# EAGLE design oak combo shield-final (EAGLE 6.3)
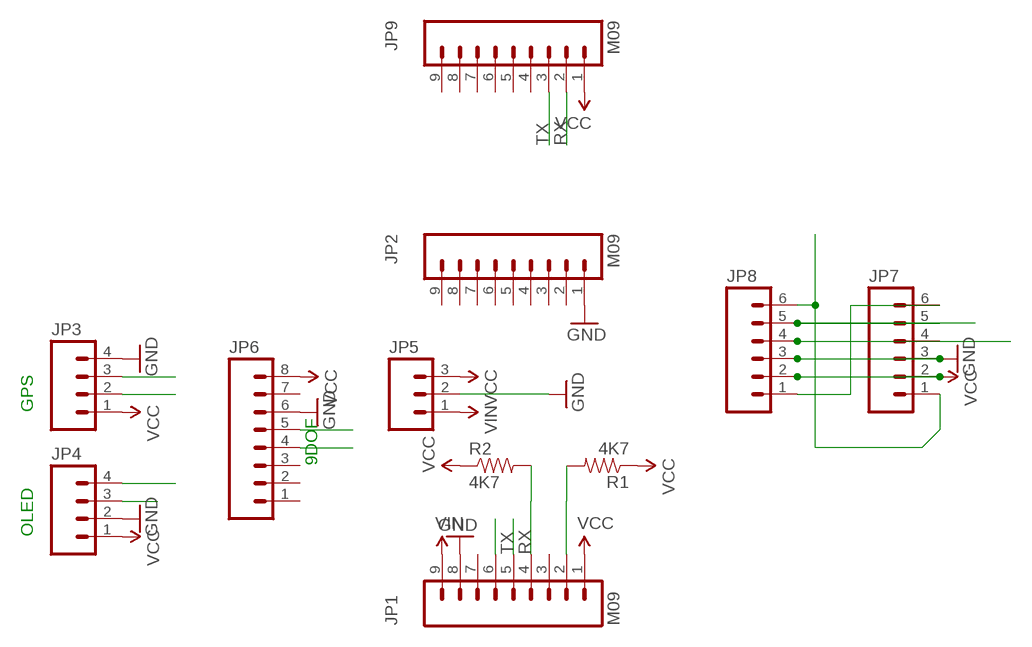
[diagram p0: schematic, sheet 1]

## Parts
JP1  M09  [1X09]
JP2  M09  [1X09]
JP3  M04PTH  [1X04]
JP4  M04PTH  [1X04]
JP5  M03PTH  [1X03]
JP6  M081X08  [1X08]
JP7  M06LOCK  [1X06_LOCK]
JP8  M06LOCK  [1X06_LOCK]
JP9  M09  [1X09]
R1  4K7  RESISTORPTH-1/4W  [AXIAL-0.4]
R2  4K7  RESISTORPTH-1/4W  [AXIAL-0.4]

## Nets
GND [POWER]: JP1.8 JP2.1 JP3.4 JP4.2 JP5.2 JP6.6 JP7.3 JP8.3
RX: JP1.5 JP3.3 JP7.4 JP8.4 JP9.2
SCL: JP1.4 JP4.3 JP6.5 R2.P$2
SDA: JP1.2 JP4.4 JP6.4 R1.P$2
STATE: JP7.1 JP8.6
TX: JP1.6 JP3.2 JP7.5 JP8.5 JP9.3
VCC: JP1.1 JP3.1 JP4.1 JP5.3 JP6.8 JP7.2 JP8.2 JP9.1 R1.P$1 R2.P$1
VIN: JP1.9 JP5.1
WAKE: JP7.6 JP8.1
Unconnected: JP1.3 JP1.7 JP2.2 JP2.3 JP2.4 JP2.5 JP2.6 JP2.7 JP2.8 JP2.9 JP6.1 JP6.2 JP6.3 JP6.7 JP9.4 JP9.5 JP9.6 JP9.7 JP9.8 JP9.9

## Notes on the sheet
- GPS
- 9DOF
- OLED

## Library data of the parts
JP1 JP2 JP9 = SparkFun:M09: Header 9 Standard 9-pin 0.1" header. Use with straight break away headers (SKU : PRT-00116), right angle break away headers (PRT-00553), swiss pins (PRT-00743), machine pins (PRT-00117), and female headers (PRT-00115).
JP3 JP4 = SparkFun-Connectors:M04: Header 4 Standard 4-pin 0.1" header. Use with straight break away headers (SKU : PRT-00116), right angle break away headers (PRT-00553), swiss pins (PRT-00743), machine pins (PRT-00117), and female headers (PRT-00115). Molex polarized connector foot print use with SKU : PRT-08231 with associated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
JP5 = SparkFun:M03: Header 3 Standard 3-pin 0.1" header. Use with straight break away headers (SKU : PRT-00116), right angle break away headers (PRT-00553), swiss pins (PRT-00743), machine pins (PRT-00117), and female headers (PRT-00115). Molex polarized connector foot print use with SKU : PRT-08232 with associated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
JP6 = SparkFun:M08: Header 8 Standard 8-pin 0.1" header. Use with straight break away headers (SKU : PRT-00116), right angle break away headers (PRT-00553), swiss pins (PRT-00743), machine pins (PRT-00117), and female headers (PRT-00115).
JP7 JP8 = SparkFun-Connectors:M06: Header 6 Standard 6-pin 0.1" header. Use with straight break away headers (SKU : PRT-00116), right angle break away headers (PRT-00553), swiss pins (PRT-00743), machine pins (PRT-00117), and female headers (PRT-00115). Molex polarized connector foot print use with SKU : PRT-08094 with associated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
R1 R2 = SparkFun-Resistors:RESISTOR: Resistor

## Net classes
1 POWER: width 0.203 mm

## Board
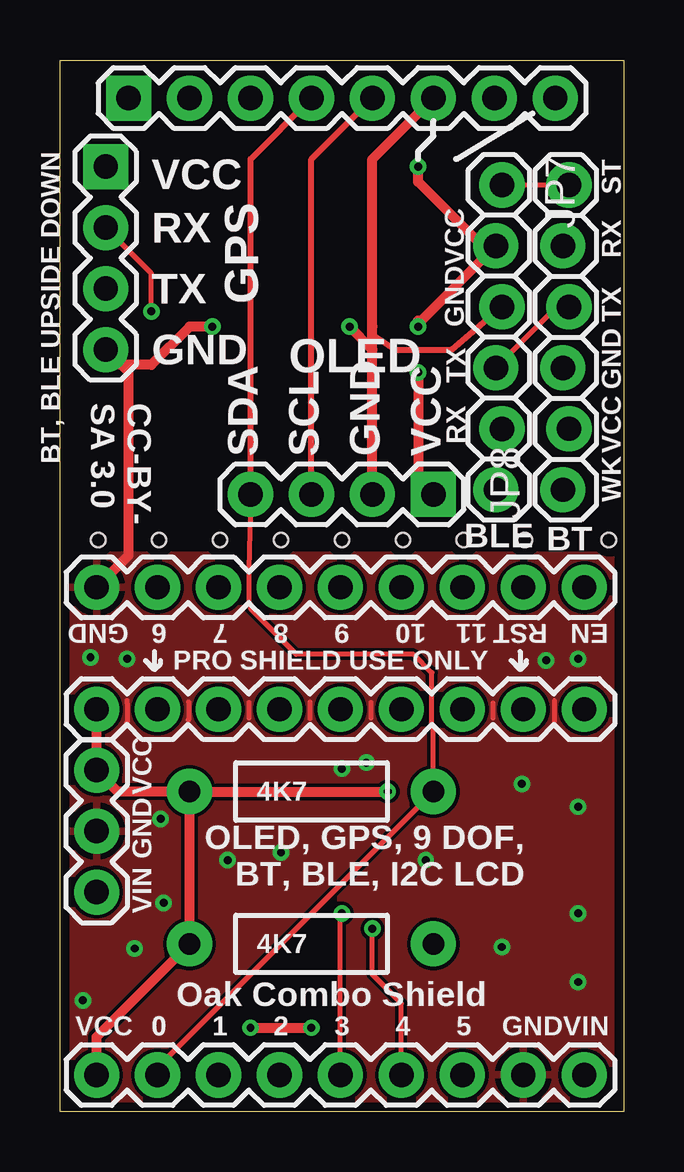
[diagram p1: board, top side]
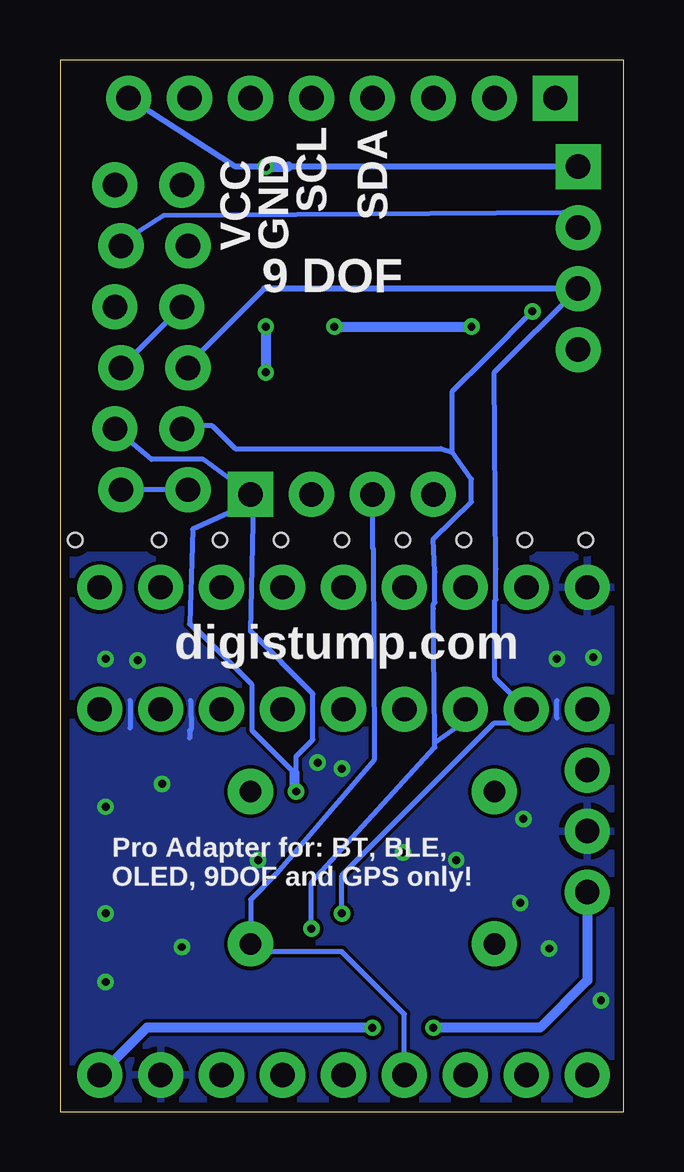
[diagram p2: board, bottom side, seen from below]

Size 23.5 x 43.81 mm. Coordinates in mm from the lower left corner, seen from the top.
Outline: 0,0 0,43.81 23.5,43.81 23.5,0 0,0
Copper layers (1*16): Top 0.0356mm / dielectric 1.5011mm / Bottom 0.0356mm
Design rules "eriks *": minimum track width 6mil, minimum drill 13mil, track to track 6mil, track to pad 8mil, pad to pad 6mil, via to via 6mil, smd to smd 6mil, copper to edge 15mil, drill to drill 6mil, minimum pad ring 7mil, minimum via ring 7mil, stop-mask expansion 4mil, vias tented up to drill 20mil, thermal gap 10mil
Holes 0.6 mm at 1.59,23.81 4.13,23.81 6.67,23.81 9.21,23.81 11.75,23.81 14.29,23.81 16.83,23.81 19.37,23.81 22.86,23.81

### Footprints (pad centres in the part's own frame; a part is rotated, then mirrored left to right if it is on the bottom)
1X09 = drill 1.016 pad 1.88: 1 0,0; 2 2.54,0; 3 5.08,0; 4 7.62,0; 5 10.16,0; 6 12.7,0; 7 15.24,0; 8 17.78,0; 9 20.32,0
1X04 = drill 1.016 pad 1.88 square: 1 0,0 | drill 1.016 pad 1.88: 2 2.54,0; 3 5.08,0; 4 7.62,0
1X03 = drill 1.016 pad 1.88: 1 0,0; 2 2.54,0; 3 5.08,0
1X08 = drill 1.016 pad 1.88 square: 1 0,0 | drill 1.016 pad 1.88: 2 2.54,0; 3 5.08,0; 4 7.62,0; 5 10.16,0; 6 12.7,0; 7 15.24,0; 8 17.78,0
1X06_LOCK = drill 1.016 pad 1.88: 1 0,0; 2 2.54,-0.254; 3 5.08,0; 4 7.62,-0.254; 5 10.16,0; 6 12.7,-0.254
AXIAL-0.4 = drill 0.9 pad 1.88: P$1 -5.08,0; P$2 5.08,0

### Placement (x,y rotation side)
JP1  1.52,1.52 0 top
JP2  1.52,21.84 0 top
JP3  1.91,39.37 270 top
JP4  15.56,25.72 180 top
JP5  1.52,9.14 90 top
JP6  2.86,42.23 0 top
JP7  18.41,38.61 270 top
JP8  20.95,25.91 90 top
JP9  1.52,16.76 0 top
R1  10.48,13.34 0 top
R2  10.48,6.99 0 top

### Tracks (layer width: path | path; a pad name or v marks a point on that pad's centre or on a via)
GND  (via drill 0.33)
  Top 0.203: 20.6,17.12 20.6,16.28 | 18.03,17.02 18.03,16.41 | 2.77,16.2 2.79,16.23 2.79,17.02 2.79,17.12 | 5.36,17.07 5.36,16.33 5.33,16.31 | 12.95,17.04 12.95,16.41 | 10.41,17.07 10.41,16.38 | 7.87,17.04 7.87,16.41
  Top 0.254: 13.02,32.7 13.02,32.38 13.97,31.75 16.32,31.75 JP7.3
  Top 0.406: JP2.1 2.86,23.18 2.86,30.8 JP3.4 2.54,31.11 3.81,31.11 5.4,32.7 v6.35,32.7 | JP4.2 13.02,28.26 | 13.02,28.26 13.02,32.7 13.02,39.69 JP6.6 | 13.02,28.26 13.02,31.75 v12.06,32.7
  Bottom 0.203: JP7.3 JP8.3 | 20.57,17.12 20.57,15.98 | 18.06,17.12 18.03,17.09 18.03,16.46 18.03,15.94 18.1,15.88 18.1,15.56 | 2.79,16.41 2.79,17.12
  Bottom 0.406: v12.06,32.7 v6.35,32.7
  other vias: 1.27,18.92 2.79,18.86 20.26,18.8 19.24,13.65 21.59,18.86 21.59,12.7 12.76,14.54 11.75,14.29 15.24,10.48 18.41,6.86 21.59,5.4 21.59,8.26 6.99,10.48 9.21,10.79 4.19,12.19 4.32,8.7 0.95,4.64 3.11,6.79
  pour Bottom: 0,23.18 0,0 23.5,0 23.5,23.18
  pour Top: 0,23.18 0,0 23.5,0 23.5,23.18
RX  (via drill 0.33)
  Top 0.203: JP1.5 11.68,8.19 v11.75,8.26 | JP8.4 20.7,33.53 JP7.4
  Bottom 0.203: v11.75,8.26 11.75,9.84 5.4,16.19 4.64,16.19 JP9.2 5.4,18.1 5.4,21.27 5.33,21.34 5.33,22.61 5.4,30.8 JP3.3 | JP7.4 18.16,31.11 14.99,34.29
  Bottom 0.254: JP3.3 14.99,34.29
SCL
  Top 0.254: JP4.3 10.48,39.69 JP6.5
  Bottom 0.203: JP4.3 10.48,23.48 10.44,23.44 10.4,14.66 14.48,9.91 15.56,8.83 R2.P$2 15.24,6.67 11.75,6.67 9.14,4.06 JP1.4
SDA
  Top 0.203: JP4.4 7.87,22.61 7.87,21.21 7.94,21.14 7.94,20.95 9.84,19.05 14.73,19.05 15.49,18.29 15.49,16.13 15.56,16.07 R1.P$2 4.06,1.84 JP1.2
  Top 0.254: JP4.4 7.94,39.69 JP6.4
STATE
  Top 0.203: JP7.1 JP8.6
TX  (via drill 0.33)
  Top 0.203: v3.81,33.34 3.81,34.92 JP3.2 | JP1.6 14.22,4.51 13.02,5.71 v13.02,7.62
  Bottom 0.203: 2.54,37.47 JP3.2 2.54,37.47 | 7.14,27.46 7.62,27.62 16.19,27.62 17.14,28.57 18.29,28.57 JP7.5 | 7.14,27.46 7.14,30 5.71,31.43 v3.81,33.34 | v13.02,7.62 13.02,9.53 7.87,15.18 7.87,15.37 | 7.87,15.37 7.87,15.68 7.94,20.95 7.94,21.14 7.87,21.21 7.87,22.48 7.94,23.88 6.35,25.4 6.35,26.35 7.14,27.46 | JP9.3 6.6,16.26 7.87,15.37 | JP8.5 20.95,36.2 19.18,37.34 2.54,37.47
VCC  (via drill 0.33)
  Top 0.254: 14.92,32.96 15.05,32.96
  Top 0.406: JP1.1 1.52,3.11 R2.P$1 R1.P$1 | R1.P$1 2.41,13.34 JP5.3 JP9.1 | R1.P$1 v13.65,13.34 | 14.92,32.96 v14.92,32.7 | v14.92,30.8 14.92,26.35 JP4.1 | 15.05,32.96 JP7.2 17.59,36.07 14.92,38.73 v14.92,39.37
  Bottom 0.203: 15.43,25.4 15.56,20 12.95,17.4 12.95,15.49 13.65,14.8 v13.65,13.34 | 15.43,25.4 JP4.1 | JP4.1 15.43,25.4 | 15.43,25.4 17.97,24.26 18.1,20.32 17.78,20 17.78,20.07 15.49,17.78 15.49,15.88 13.72,14.1 | JP4.1 17.53,27.18 19.68,27.18 JP8.2
  Bottom 0.254: JP3.1 13.97,39.37 v14.92,39.37 16.19,39.37 JP6.8
  Bottom 0.406: v14.92,32.7 v14.92,30.8 | 13.72,13.34 13.72,14.1 | v14.92,39.37 13.97,39.37
VIN  (via drill 0.33)
  Top 0.406: v7.94,3.49 v10.48,3.49
  Bottom 0.406: JP5.1 1.52,5.46 3.49,3.49 v7.94,3.49 | v10.48,3.49 19.88,3.49 JP1.9
WAKE
  Bottom 0.203: JP7.6 JP8.1

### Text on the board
tPlace: VCC | ST | RX | RX | VCC | TX | GPS | GND | TX | GND | OLED | CC-BY- / SA 3.0 | TX | GND | RX | BT, BLE UPSIDE DOWN | SDA | SCL | GND | VCC | VCC | WK | BLE | BT | GND | 6 | 7 | 8 | 9 | 10 | 11 | RST | EN | PRO SHIELD USE ONLY | VCC | OLED, GPS, 9 DOF, / BT, BLE, I2C LCD | GND | VIN | Oak Combo Shield | VCC | 0 | 0 | 1 | 2 | 3 | 4 | 5 | GND | VIN
bPlace: SDA | SCL | 9 DOF | GND | VCC | digistump.com | Pro Adapter for: BT, BLE, / OLED, 9DOF and GPS only!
